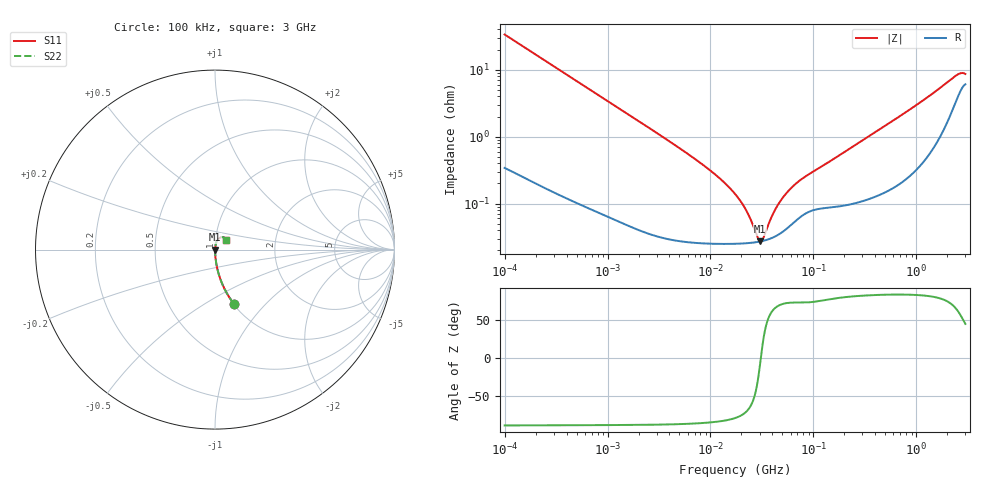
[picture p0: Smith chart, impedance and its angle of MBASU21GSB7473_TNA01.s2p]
! MBASU21GSB7473_TNA01  S-PARAMETER MODEL  ( Standard Model )
! Model Generated by TAIYO YUDEN Corporation (http://www.ty-top.com)
! Version 1.0
! TAIYO YUDEN Control No. 220601
! Copyright(c) 2012 TAIYO YUDEN CO.,LTD. All Rights Reserved.
! Product Description (link to TY-COMPAS)
! https://ds.yuden.co.jp/TYCOMPAS/or/detail?pn=MBASU21GSB7473KTNA01&u=M
! Products Name : Multilayer Ceramic Capacitors
! Characteristics :
!  Capacitance : 0.047 [uF] , Rated Voltage : 50 [V] , TCC : X7R
!  Case Size : 2.0 x 1.25 / 0.079 x 0.049 [mm/inch] , Thickness : 1.25 / 0.049 [mm/inch]
!  (Conditions: Temperature = 25 [degC] , DC Bias Voltage = 0 [V])
! External Node Assignments :
!  1  o---| |---o  2
! GND o---------o GND
! Frequency Range : 100kHz  -  3GHz  [ 401 STEP ]
# MHZ S RI R 50
! Freq[MHz].  S11 Real  S11 Imag  S21 Real  S21 Imag  S12 Real  S12 Imag  S22 Real  S22 Imag
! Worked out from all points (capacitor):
!   401 points, 100 kHz to 3 GHz, reference 50 ohm
!   read as one part in series: C = 47.2 nF near 105.3 kHz
!   lowest |Z| = 27.3 mohm at 30.54 MHz (marker M1)
!   series resonance near 30.86 MHz, so ESL is about 560 pH
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0.1  0.1041 -0.3004  0.8959 0.3004  0.8959 0.3004  0.1041 -0.3004
0.228123  0.0232 -0.1446  0.9768 0.1446  0.9768 0.1446  0.0232 -0.1446
0.562235  0.00459 -0.0602  0.9954 0.0602  0.9954 0.0602  0.00459 -0.0602
3.161081  0.000435 -0.0108  0.9996 0.0108  0.9996 0.0108  0.000435 -0.0108
9.824692  0.000262 -0.00317  0.9997 0.00317  0.9997 0.00317  0.000262 -0.00317
13.7349  0.000254 -0.00203  0.9997 0.00203  0.9997 0.00203  0.000254 -0.00203
17.7727  0.000253 -0.00131  0.9997 0.00131  0.9997 0.00131  0.000253 -0.00131
22.41241  0.000257 -0.000736  0.9997 0.000736  0.9997 0.000736  0.000257 -0.000736
24.84619  0.00026 -0.000495  0.9997 0.000495  0.9997 0.000495  0.00026 -0.000495
28.26337  0.000267 -0.0002  0.9997 0.0002  0.9997 0.0002  0.000267 -0.0002
30.53531  0.000272 -2.42e-05  0.9997 2.42e-05  0.9997 2.42e-05  0.000272 -2.42e-05
32.98988  0.00028 0.000152  0.9997 -0.000152  0.9997 -0.000152  0.00028 0.000152
40.54368  0.000312 0.000631  0.9997 -0.000631  0.9997 -0.000631  0.000312 0.000631
44.94634  0.000339 0.000879  0.9997 -0.000879  0.9997 -0.000879  0.000339 0.000879
51.12795  0.000387 0.0012  0.9996 -0.0012  0.9996 -0.0012  0.000387 0.0012
67.88584  0.000562 0.00192  0.9994 -0.00192  0.9994 -0.00192  0.000562 0.00192
97.38194  0.000795 0.00284  0.9992 -0.00284  0.9992 -0.00284  0.000795 0.00284
547.5153  0.00183 0.0159  0.9982 -0.0159  0.9982 -0.0159  0.00183 0.0159
1535  0.00961 0.046  0.9904 -0.046  0.9904 -0.046  0.00961 0.046
2378.954  0.035 0.0691  0.965 -0.0691  0.965 -0.0691  0.035 0.0691
2706.139  0.0516 0.0669  0.9484 -0.0669  0.9484 -0.0669  0.0516 0.0669
3000  0.0603 0.0545  0.9397 -0.0545  0.9397 -0.0545  0.0603 0.0545
